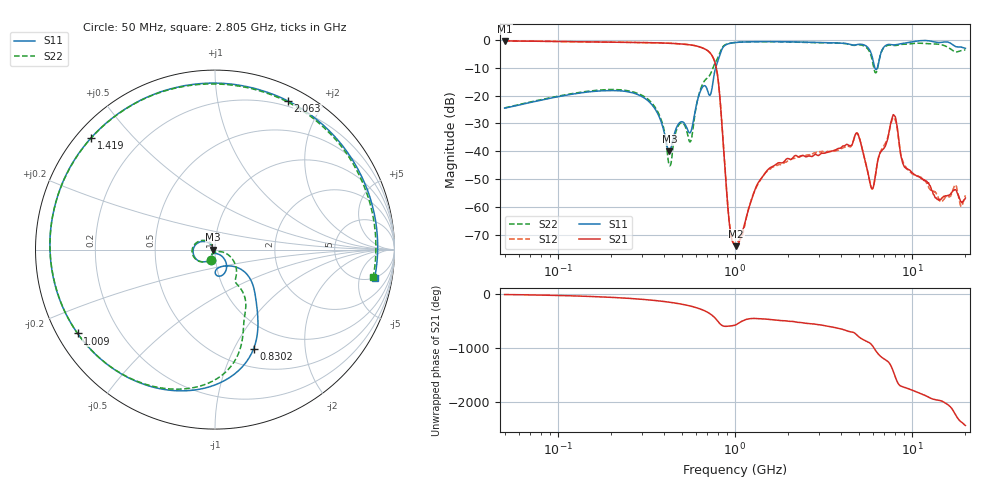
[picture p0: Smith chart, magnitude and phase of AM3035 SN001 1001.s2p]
# Hz S DB R 50
!freq MagS11 AngS11 MagS21 AngS21 MagS12 AngS12 MagS22 AngS22
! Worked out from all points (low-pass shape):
!   1601 points, 50 MHz to 20.05 GHz, reference 50 ohm
!   highest |S21| = -0.36 dB at 50 MHz (marker M1); lowest = -74.1 dB at 1.016 GHz (marker M2)
!   |S21| within 3 dB of the highest: start of sweep to 681.1 MHz
!   lowest |S11| = -40.0 dB at 426.2 MHz (marker M3), VSWR 1.02, Z = 49 - j0.126 ohm
!   |S11| at or under -10 dB: start of sweep to 778.2 MHz; 6.176 GHz to 6.38 GHz (204.2 MHz wide, 3.25 % of centre)
!   |S22| runs from -45.2 to -0.6 dB; largest |S21 - S12| = 0.006
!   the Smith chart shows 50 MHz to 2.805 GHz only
!   S11 on the Smith chart (normalised r, x): 50 MHz: 0.95, -0.11; 830.2 MHz: 0.71, -1.20; 1.009 GHz: 0.06, -0.28; 1.419 GHz: 0.04, +0.38; 2.063 GHz: 0.14, +1.60; 2.805 GHz: 4.81, -8.44
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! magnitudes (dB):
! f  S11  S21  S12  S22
! 50 MHz  -24.5  -0.4  -0.4  -24.4
! 135.9 MHz  -19.0  -0.7  -0.7  -18.7
! 369.6 MHz  -27.0  -1.1  -1.1  -26.3
! 426.2 MHz  -40.0  -1.2  -1.2  -45.0
! 562.3 MHz  -33.1  -1.8  -1.8  -36.4
! 725.5 MHz  -19.8  -4.7  -4.7  -12.4
! 830.2 MHz  -4.6  -23.9  -23.8  -4.0
! 929 MHz  -1.3  -65.6  -65.3  -1.2
! 1.005 GHz  -1.0  -73.8  -73.1  -0.9
! 1.009 GHz  -0.9  -73.9  -73.1  -0.9
! 1.016 GHz  -0.9  -74.1  -73.0  -0.9
! 1.419 GHz  -0.6  -49.6  -49.5  -0.6
! 2.063 GHz  -0.7  -42.9  -43.0  -0.8
! 2.722 GHz  -0.9  -41.9  -41.1  -1.0
! 2.805 GHz  -0.9  -41.3  -40.6  -1.0
! 4.902 GHz  -1.7  -33.5  -33.4  -1.8
! 5.956 GHz  -5.9  -53.5  -53.5  -7.1
! 7.402 GHz  -1.6  -33.5  -33.6  -1.9
! 7.978 GHz  -1.8  -27.3  -28.1  -2.1
! 9.061 GHz  -1.2  -45.5  -44.9  -1.6
! 14.47 GHz  -0.9  -57.3  -58.0  -1.7
! 20.05 GHz  -3.0  -56.8  -55.8  -3.6
